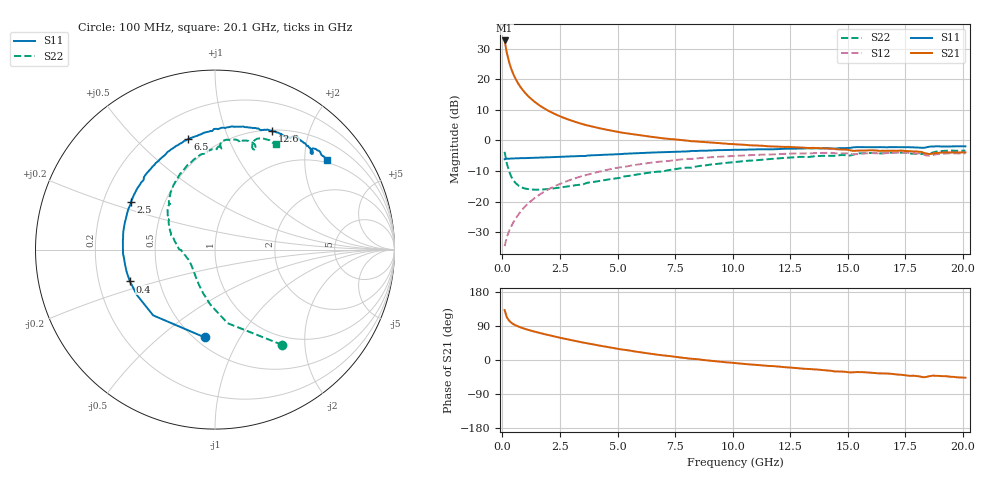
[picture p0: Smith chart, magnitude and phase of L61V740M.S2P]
!  Infineon Technologies AG
! BFR380L3 , PF131585-7, No.6, Th 09.10.01, soldered on pcb-board, measured with PP GSG850
!  Vce=1.75 V,  Ic=40.0 mA
! Common Emitter S-Parameters:  15. November 2001
#  GHz  S  MA  R  50
! f  S11  S21  S12  S22
! GHz  Mag  Ang  Mag  Ang  Mag  Ang  Mag  Ang
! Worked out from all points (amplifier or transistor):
!   201 points, 100 MHz to 20.1 GHz, reference 50 ohm
!   highest |S21| = 32.7 dB at 100 MHz (marker M1)
!   |S21| within 3 dB of that: start of sweep to 171.8 MHz
!   unconditionally stable (mu >= 1): 987.8 MHz to 4.35 GHz
!   at 3.4 GHz: K = 1.02, MAG = 7.9 dB, |S12| = -11.8 dB
!   at 10.1 GHz: K = 0.96, MSG = 1.9 dB, |S12| = -5.1 dB
!   at 20.1 GHz: K = 0.99, MSG = 0.1 dB, |S12| = -4.2 dB
!   S11 on the Smith chart (normalised r, x): 100 MHz: 0.56, -0.72; 400 MHz: 0.34, -0.16; 2.5 GHz: 0.32, +0.24; 6.5 GHz: 0.35, +0.72; 12.6 GHz: 0.51, +1.46; 20.1 GHz: 0.93, +2.55
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0.1  0.4926 -96.6  43.04 131.8  0.01866 59.1  0.6498 -54.8
0.2  0.5029 -133.2  26.6 112.3  0.02652 57.4  0.4159 -80.3
0.3  0.5033 -149.8  18.73 103.4  0.03344 59.6  0.3072 -94.9
0.4  0.5062 -159.5  14.35 97.9  0.04018 62.1  0.2504 -105.5
0.5  0.5076 -165.6  11.6 93.9  0.04724 64.4  0.2174 -113.9
0.6  0.5083 -170.5  9.741 90.9  0.05434 66.0  0.1968 -120.8
0.7  0.509 -174.4  8.389 88.2  0.06149 67.0  0.183 -126.6
0.8  0.5132 -177.6  7.364 85.9  0.06911 67.8  0.1737 -131.6
1  0.5137 177.0  5.931 81.8  0.08394 68.4  0.163 -139.7
1.3  0.5191 170.4  4.6 76.5  0.1064 68.3  0.1571 -148.5
1.6  0.523 164.6  3.767 71.7  0.1287 67.3  0.1566 -155.1
2  0.5294 157.8  3.05 65.7  0.1583 65.3  0.1604 -162.0
2.5  0.5386 150.2  2.482 58.8  0.1942 62.3  0.1689 -168.9
3.5  0.5558 136.3  1.839 46.1  0.2638 55.4  0.1907 -179.7
4.9  0.5921 119.9  1.404 30.7  0.3507 45.2  0.2386 165.0
6.5  0.633 104.0  1.141 15.9  0.4347 33.6  0.3009 149.1
6.8  0.6381 101.2  1.102 13.5  0.4479 31.3  0.309 146.0
10.1  0.7034 77.2  0.8634 -8.1  0.5587 9.7  0.4437 119.1
12.6  0.7319 64.4  0.7745 -20.4  0.6096 -5.3  0.5269 100.2
13.5  0.7397 60.1  0.7547 -24.6  0.6175 -10.4  0.546 94.6
16.8  0.7763 48.1  0.6794 -36.0  0.6223 -25.8  0.628 75.2
20.1  0.7982 38.7  0.6357 -46.8  0.6163 -39.1  0.6816 60.0
